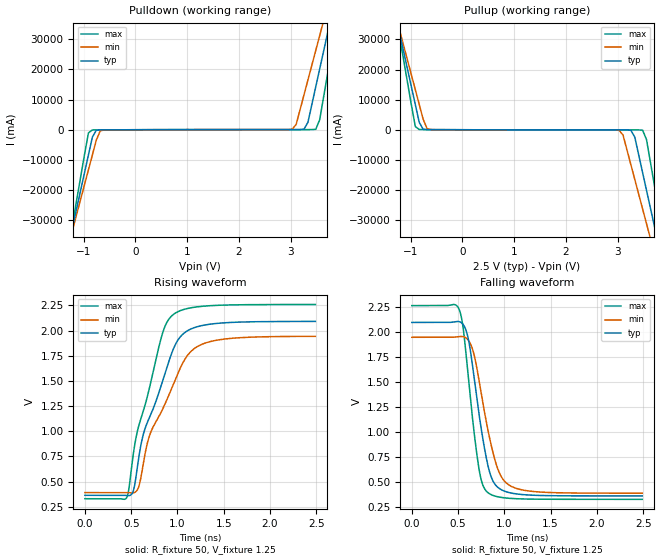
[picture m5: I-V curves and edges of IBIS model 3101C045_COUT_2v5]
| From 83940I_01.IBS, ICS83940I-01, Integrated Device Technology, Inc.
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[Model] 3101C045_COUT_2v5
Model_type  Output
Polarity   Non-Inverting
Vmeas = 1.25
Rref = 50
Cref = 0
Vref = 1.25
|Variable  typ   min   max
C_comp   2p   1.5p   2.5p
[Voltage Range]   2.5   2.375   2.625
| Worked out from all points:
|   slope of the pulldown table from 0 to 0.375 V, typ, clamps not added: 20.7 ohm
|   slope of the pullup table from 0 to 0.375 V, typ, clamps not added: 24 ohm
|   rising waveform, R_fixture 50, V_fixture 1.25: 20-80 % time 349ps typ, 398ps min, 294ps max; typ from 0.364 V to 2.09 V
|   falling waveform, R_fixture 50, V_fixture 1.25: 20-80 % time 169ps typ, 201ps min, 137ps max; typ from 2.09 V to 0.364 V
| Open source, no load
|  Voltage   I(typ)   I(min)   I(max)
[Pullup]
-2.5V     132.3A     116.5A     159.2A
-1.288V   37.85A     37.86A     38.39A
-1.212V   31.95A     32.95A     30.84A
-909.1mV  8.343A     13.29A     1.049A
-833.3mV  2.441A     8.379A     73.62mA
-606.1mV  30.67mA    56.76mA    36.71mA
3.03V     -45.63mA   -189.1mA   -56.57mA
3.333V    -2.451A    -16.49A    -59.61mA
3.485V    -14.25A    -26.32A    -150.7mA
3.712V    -31.96A    -41.06A    -18.4A
3.864V    -43.76A    -50.88A    -33.49A
5V        -132.3A    -124.6A    -146.7A
[Pulldown]
-2.5V     -132.3A    -116.5A    -159.1A
-1.288V   -37.86A    -37.86A    -38.39A
-1.212V   -31.95A    -32.95A    -30.84A
-909.1mV  -8.345A    -13.29A    -1.048A
-833.3mV  -2.443A    -8.38A     -72.91mA
-606.1mV  -31.63mA   -57.75mA   -36.23mA
3.03V     41.73mA    184.6mA    49.3mA
3.333V    2.442A     16.48A     49.69mA
3.485V    14.24A     26.3A      135.8mA
3.712V    31.94A     41.04A     18.38A
3.864V    43.74A     50.86A     33.46A
5V        132.3A     124.6A     146.6A
[Ramp]
|   typ   min   max
dV/dt_r   1.384/0.464n   1.243/0.534n   1.548/0.388n
dV/dt_f   1.389/0.253n   1.248/0.307n   1.551/0.201n
R_load =   50.0000
[Rising Waveform]
R_fixture = 50
V_fixture = 1.25   | VCC_typ
V_fixture_max = 1.3125   | VCC_max
V_fixture_min = 1.1875   | VCC_min
C_fixture = 0.0p
| Time   typ   min   max
0s        364.1mV    391.2mV    330mV
454.5ps   361.1mV    391.2mV    346.8mV
522ps     406.2mV    388.8mV    767.6mV
571.9ps   678mV      427mV      1.02V
699.3ps   1.14V      959.8mV    1.438V
841.7ps   1.505V     1.224V     1.982V
949.1ps   1.802V     1.452V     2.155V
1.109ns   1.999V     1.754V     2.219V
1.296ns   2.055V     1.875V     2.243V
2.49ns    2.091V     1.943V     2.259V
[Falling Waveform]
R_fixture = 50
V_fixture = 1.25   | VCC_typ
V_fixture_max = 1.3125   | VCC_max
V_fixture_min = 1.1875   | VCC_min
C_fixture = 0.0p
| Time   typ   min   max
0s        2.091V     1.944V     2.259V
512ps     2.099V     1.951V     2.22V
554.4ps   2.072V     1.95V      2.039V
609.4ps   1.933V     1.915V     1.556V
664.3ps   1.604V     1.8V       1.068V
721.8ps   1.209V     1.54V      657.9mV
821.7ps   670.6mV    1.024V     397.3mV
946.6ps   437.3mV    593mV      352.2mV
1.099ns   388.4mV    449.3mV    337.5mV
2.49ns    364.1mV    391.2mV    330mV
